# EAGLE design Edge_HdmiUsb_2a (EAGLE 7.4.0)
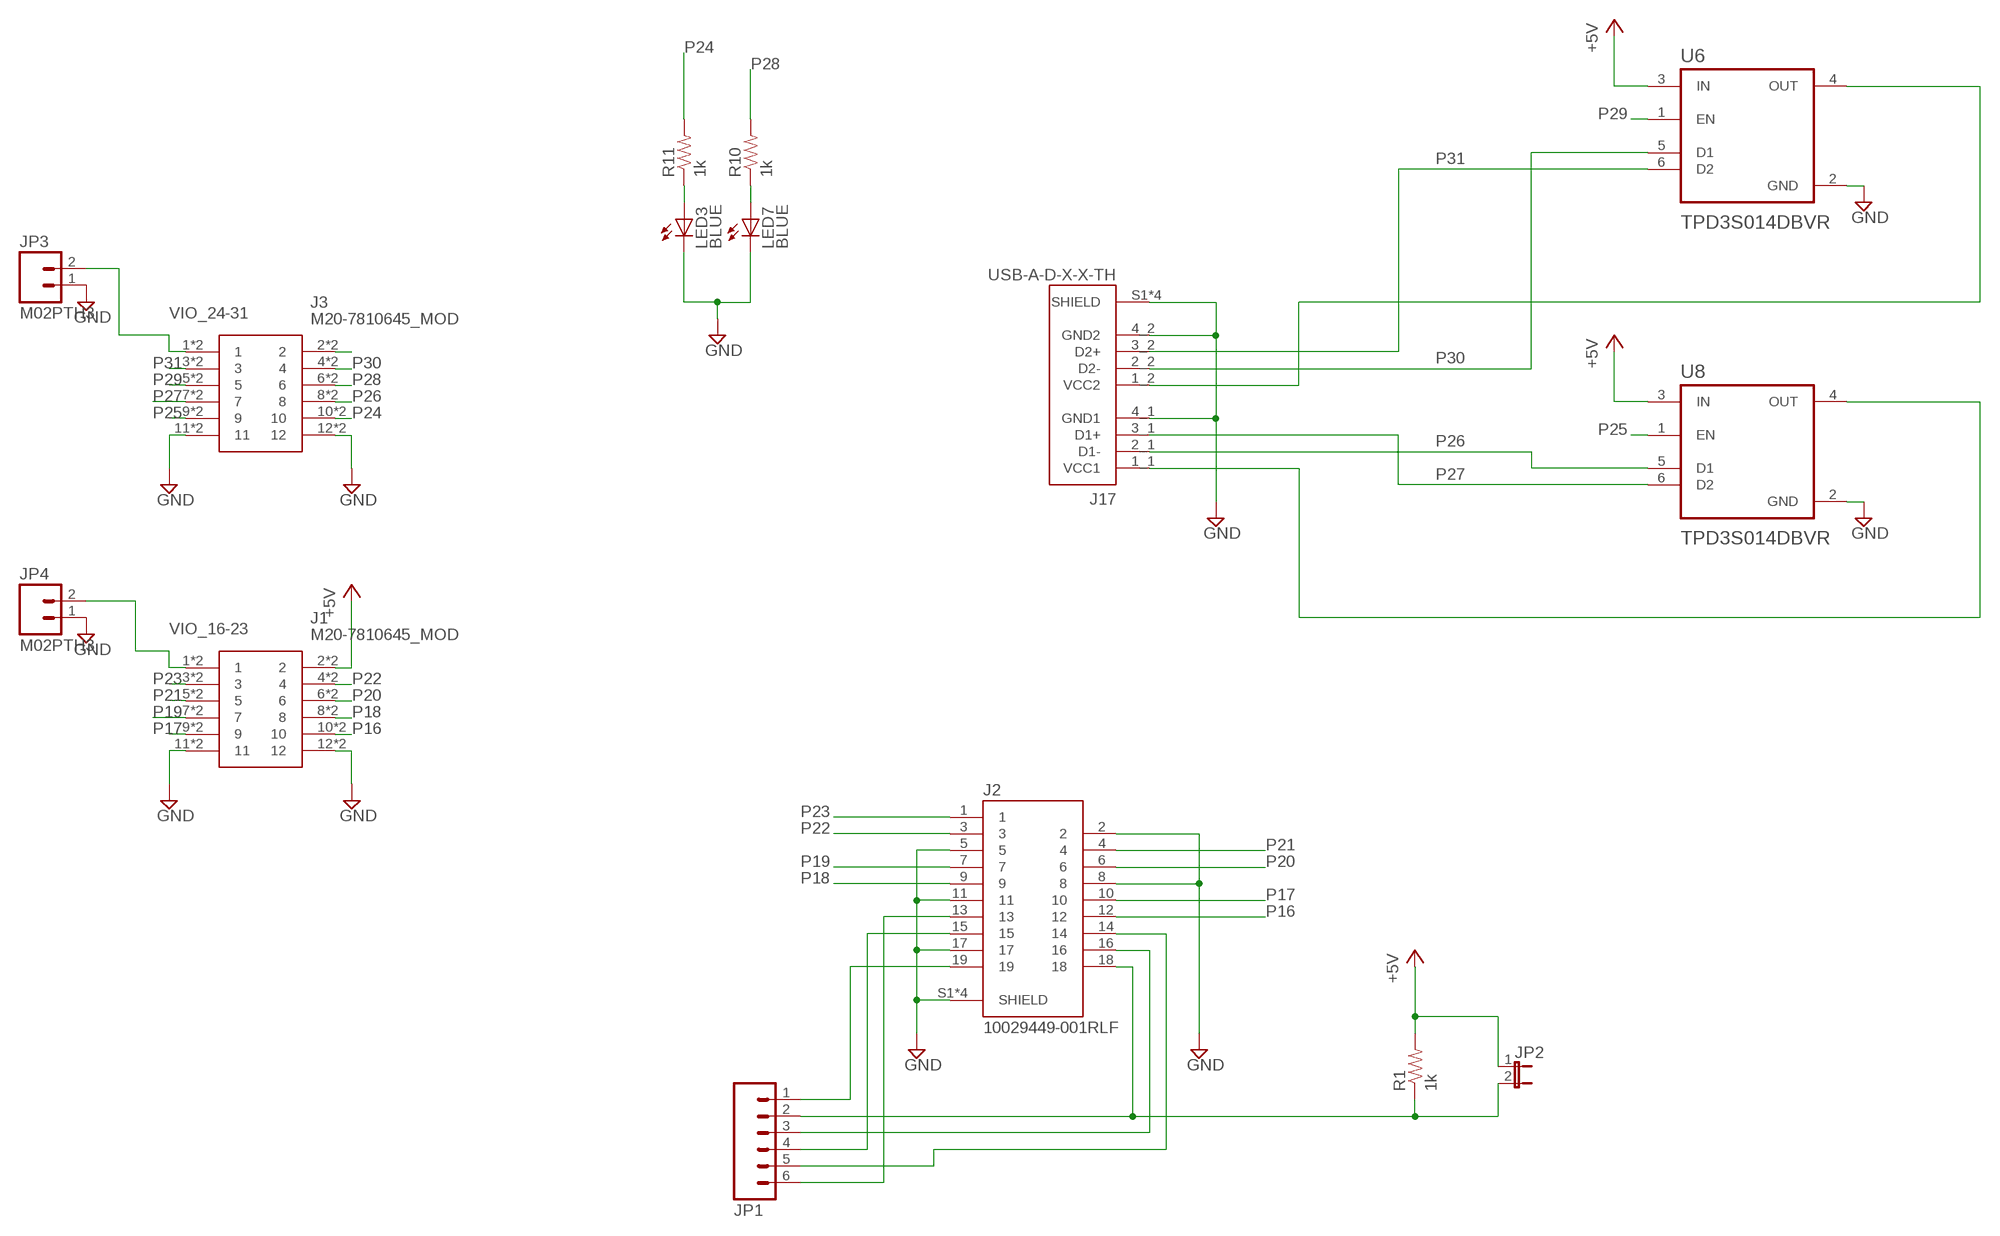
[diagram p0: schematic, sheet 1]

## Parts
J1  M20-7810645_MOD  [M207810645_MOD]
J2  10029449-001RLF  [AMPHENOL_10029449-001RLF]
J3  M20-7810645_MOD  [M207810645_MOD]
J17  USB-A-D-X-X-TH  [SAMTEC_USB-A-D-X-X-TH]
JP1  M06SIP  [1X06]
JP2  JUMPER-2SMD-NO  [SJ_2S-NO]
JP3  M02PTH3  [1X02_LONGPADS]
JP4  M02PTH3  [1X02_LONGPADS]
LED3  BLUE  LEDSML0805  [SML0805]
LED7  BLUE  LEDSML0805  [SML0805]
R1  1k  0.75OHM1/4W1%(0805)  [0805]
R10  1k  0.75OHM1/4W1%(0805)  [0805]
R11  1k  0.75OHM1/4W1%(0805)  [0805]
U6  TPD3S014DBVR  [SOT95P280X145-6N]
U8  TPD3S014DBVR  [SOT95P280X145-6N]

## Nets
+5V: J1.2 J1.2A JP2.1 R1.2 U6.3(IN) U8.3(IN)
GND [power]: J1.11 J1.11A J1.12 J1.12A J2.2 J2.5 J2.8 J2.11 J2.17 J2.S1(SHIELD) J2.S2(SHIELD) J2.S3(SHIELD) J2.S4(SHIELD) J3.11 J3.11A J3.12 J3.12A J17.4_1(GND1) J17.4_2(GND2) J17.S1(SHIELD) J17.S2(SHIELD) J17.S3(SHIELD) J17.S4(SHIELD) JP3.1 JP4.1 LED3.C LED7.C U6.2(GND) U8.2(GND)
N$1: J2.18 JP1.2 JP2.2 R1.1
N$2: J2.16 JP1.3
N$3: J17.1_1(VCC1) U8.4(OUT)
N$4: J2.15 JP1.4
N$5: J2.14 JP1.5
N$6: J3.2 J3.2A
N$8: J2.13 JP1.6
N$19: J2.19 JP1.1
N$23: LED3.A R11.1
N$26: J17.1_2(VCC2) U6.4(OUT)
N$27: LED7.A R10.1
P16: J1.10 J1.10A J2.12
P17: J1.9 J1.9A J2.10
P18: J1.8 J1.8A J2.9
P19: J1.7 J1.7A J2.7
P20: J1.6 J1.6A J2.6
P21: J1.5 J1.5A J2.4
P22: J1.4 J1.4A J2.3
P23: J1.3 J1.3A J2.1
P24: J3.10 J3.10A R11.2
P25: J3.9 J3.9A U8.1(EN)
P26: J3.8 J3.8A J17.2_1(D1-) U8.5(D1)
P27: J3.7 J3.7A J17.3_1(D1+) U8.6(D2)
P28: J3.6 J3.6A R10.2
P29: J3.5 J3.5A U6.1(EN)
P30: J3.4 J3.4A J17.2_2(D2-) U6.5(D1)
P31: J3.3 J3.3A J17.3_2(D2+) U6.6(D2)
VIO_16-23: J1.1 J1.1A JP4.2
VIO_24-31: J3.1 J3.1A JP3.2

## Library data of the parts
J1 J3 = ray2:M20-7810645_MOD: Headers & Wire Housings 6+6 DIL 2.54MM L/P SMT SKT Source: Datasheet; DESCRIPTION: Headers & Wire Housings 6+6 DIL 2.54MM L/P SMT SKT; HEIGHT: 3.7mm; MANUFACTURER_NAME: Harwin; MANUFACTURER_PART_NUMBER: M20-7810645; MOUSER_PART_NUMBER: 855-M20-7810645; MOUSER_PRICE-STOCK: https://www.mouser.co.uk/ProductDetail/Harwin/M20-7810645?qs=k41KVqW3ympKz0jQ%252Bxdz7A%3D%3D
J2 = ray2:10029449-001RLF: Connector, Hdmi Type a, Receptacle, 19 Position, Full Ree; AVAILABILITY: Unavailable; DESCRIPTION: Connector, Hdmi Type a, Receptacle, 19 Position, Full Reel; MF: Amphenol ICC; MP: 10029449-001RLF; PACKAGE: None; PRICE: None
J17 = ray2:USB-A-D-X-X-TH: USB-A (USB TYPE-A), Stacked USB 2.0 Receptacle Connector 8 Position Through Hole, Right Angle Check availability; AVAILABILITY: In Stock; DESCRIPTION: USB-A (USB TYPE-A), Stacked USB 2.0 Receptacle Connector 8 Position Through Hole, Right Angle; MF: Samtec; MP: USB-A-D-F-B-TH; PACKAGE: None; PRICE: None; PURCHASE-URL: https://pricing.snapeda.com/search/part/USB-A-D-F-B-TH/?ref=eda
JP1 = SparkFun-Connectors:M06: Header 6 Standard 6-pin 0.1" header. Use with straight break away headers (SKU : PRT-00116), right angle break away headers (PRT-00553), swiss pins (PRT-00743), machine pins (PRT-00117), and female headers (PRT-00115). Molex polarized connector foot print use with SKU : PRT-08094 with associated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
JP2 = SparkFun-Passives:JUMPER-2: Jumper
JP3 JP4 = SparkFun-Connectors:M02: Standard 2-pin 0.1" header. Use with
LED3 LED7 = led:LED: LED
R1 R10 R11 = SparkFun-Resistors:0.75OHM1/4W1%(0805): RES-08474; PROD_ID: RES-08474; VALUE: 0.75
U6 U8 = ray2:TPD3S014DBVR: Current Limit Switch and D+/D? ESD Protection for USB Host Ports 6-SOT-23 -40 to 85; DESCRIPTION: Current Limit Switch and D+/D? ESD Protection for USB Host Ports 6-SOT-23 -40 to 85; DIGI-KEY_PART_NUMBER: 296-38835-1-ND; DIGI-KEY_PURCHASE_URL: https://www.digikey.com/product-detail/en/texas-instruments/TPD3S014DBVR/296-38835-1-ND/5138398?utm_source=snapeda&utm_medium=aggregator&utm_campaign=symbol; MF: Texas Instruments; MP: TPD3S014DBVR; PACKAGE: SOT-23-6 Texas Instruments

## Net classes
1 power: width 0.254 mm

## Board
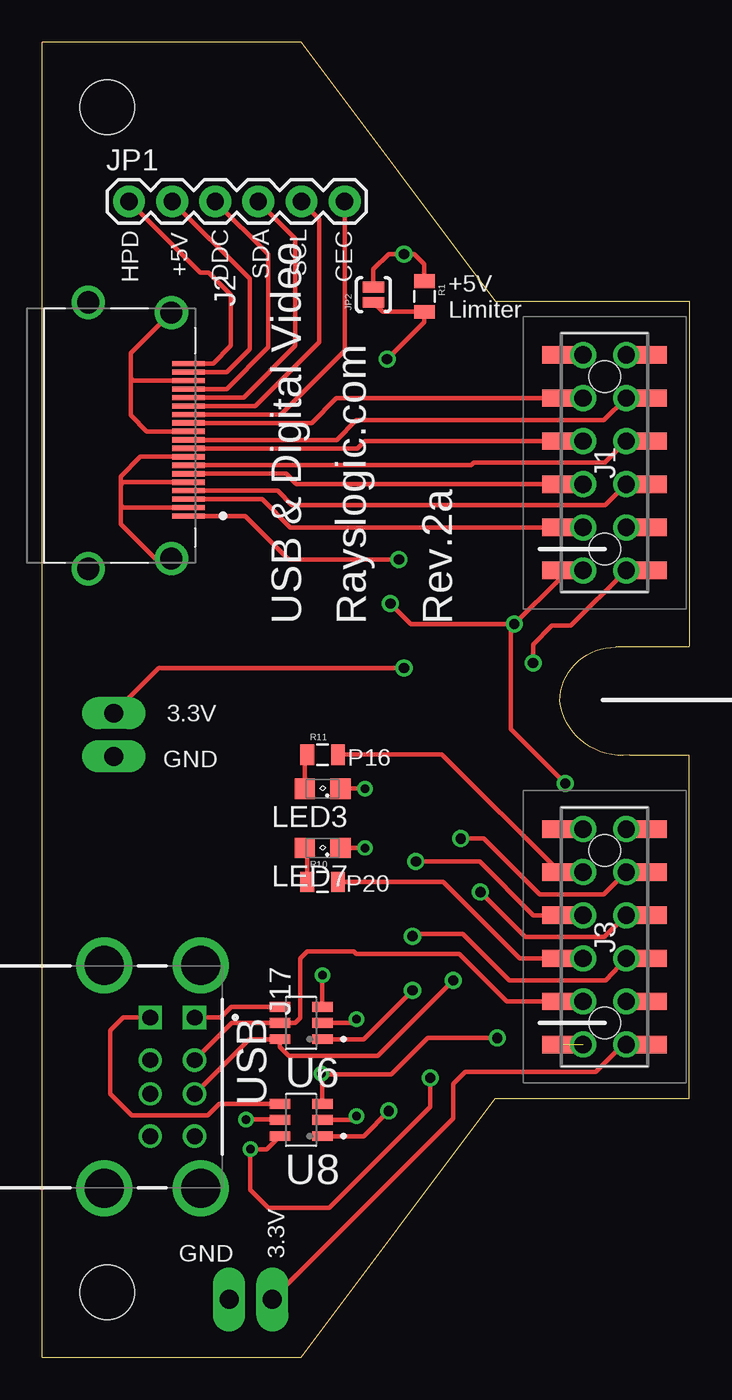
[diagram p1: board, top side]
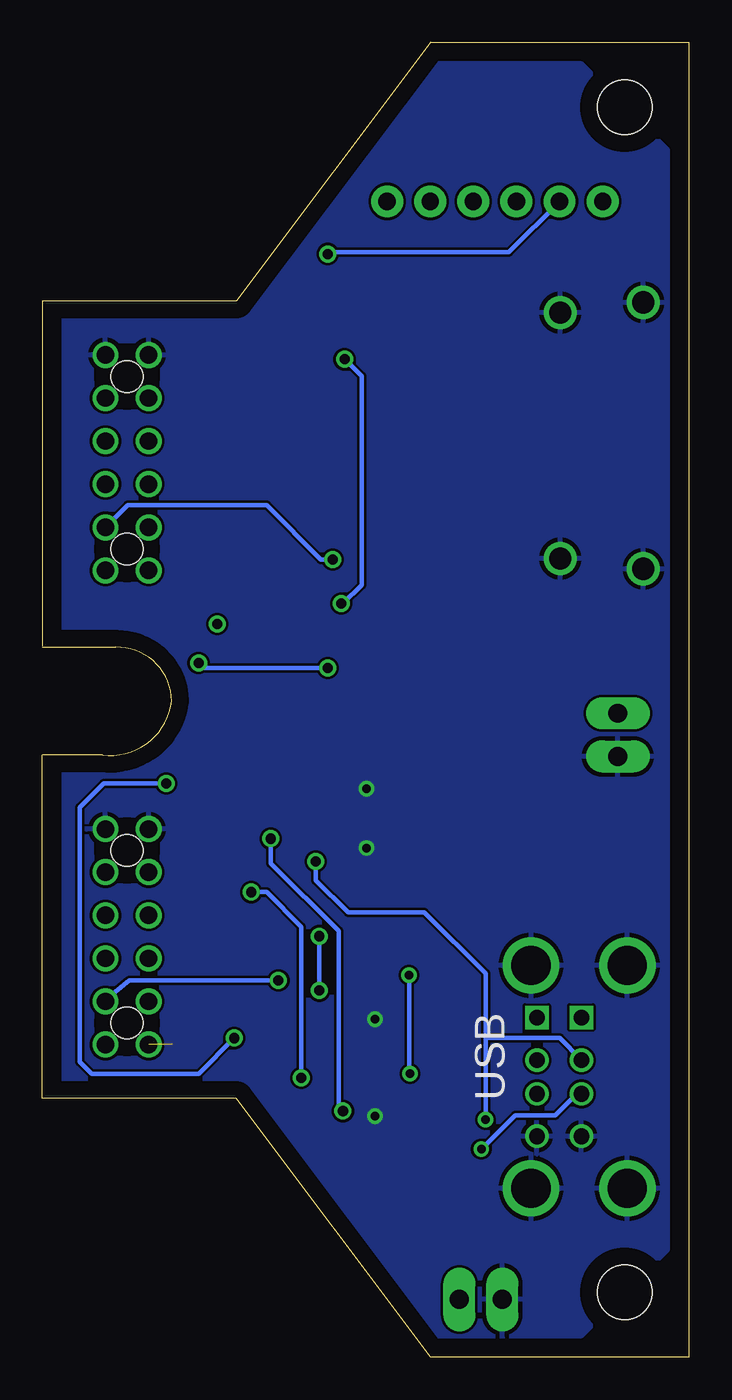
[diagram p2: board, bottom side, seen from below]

Size 38.1 x 77.47 mm. Coordinates in mm from the lower left corner, seen from the top.
Outline: 38.1,41.84 33.78,41.84 arc90 30.48,38.66 arc90 34.56,35.48 38.1,35.48 38.1,15.24 26.67,15.24 15.24,0 0,0 0,77.47 15.24,77.47 26.67,62.23 38.1,62.23 38.1,41.91
Copper layers (1*16): Top 0.035mm / dielectric 1.5mm / Bottom 0.035mm
Design rules "default *": minimum track width 5mil, minimum drill 8mil, track to track 6mil, track to pad 6mil, pad to pad 6mil, via to via 8mil, smd to smd 8mil, copper to edge 40mil, drill to drill 8mil, minimum pad ring 4mil, minimum via ring 8mil, stop-mask expansion 4mil, vias tented up to drill 0mil, thermal gap 10mil
Holes 3.2 mm at 3.81,3.81 3.81,73.66

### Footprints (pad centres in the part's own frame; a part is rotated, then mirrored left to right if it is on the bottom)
M207810645_MOD = smd 1.02 x 2.034: 1 -6.35,-2.656; 2 -6.35,2.656; 3 -3.81,-2.656; 4 -3.81,2.656; 5 -1.27,-2.656; 6 -1.27,2.656; 7 1.27,-2.656; 8 1.27,2.656; 9 3.81,-2.656; 10 3.81,2.656; 11 6.35,-2.656; 12 6.35,2.656 | drill 1.02: 1A -6.35,-1.27; 2A -6.35,1.27; 3A -3.81,-1.27; 4A -3.81,1.27; 5A -1.27,-1.27; 6A -1.27,1.27; 7A 1.27,-1.27; 8A 1.27,1.27; 9A 3.81,-1.27; 10A 3.81,1.27; 11A 6.35,-1.27; 12A 6.35,1.27 | hole 1.85: -5.08,0; 5.08,0
AMPHENOL_10029449-001RLF = smd 0.3 x 1.9: 1 4.75,1; 2 4.25,1; 3 3.75,1; 4 3.25,1; 5 2.75,1; 6 2.25,1; 7 1.75,1; 8 1.25,1; 9 0.75,1; 10 0.25,1; 11 -0.25,1; 12 -0.75,1; 13 -1.25,1; 14 -1.75,1; 15 -2.25,1; 16 -2.75,1; 17 -3.25,1; 18 -3.75,1; 19 -4.25,1 | drill 1.3: S1 7.25,0; S2 -7.25,0; S3 -7.85,-4.9; S4 7.85,-4.9
SAMTEC_USB-A-D-X-X-TH = drill 0.92 square: 1_1 -3.5,0; 1_2 -3.5,2.62 | drill 0.92: 2_1 -1,0; 2_2 -1,2.62; 3_1 1,0; 3_2 1,2.62; 4_1 3.5,0; 4_2 3.5,2.62 | drill 2.3: S1 -6.57,2.97; S2 6.57,2.97; S3 -6.57,-2.71; S4 6.57,-2.71
1X06 = drill 1.016 pad 1.88: 1 0,0; 2 2.54,0; 3 5.08,0; 4 7.62,0; 5 10.16,0; 6 12.7,0
SJ_2S-NO = smd 0.635 x 1.27: 1 -0.45,0; 2 0.45,0
1X02_LONGPADS = drill 1.118 pad 1.88 long: 1 0,0; 2 2.54,0
SML0805 = smd 1.2 x 1.2: A 1.05,0; C -1.05,0
0805 = smd 0.8 x 1.2: 1 -0.9,0; 2 0.9,0
SOT95P280X145-6N = smd 1.21 x 0.58: 1 -1.255,0.95; 2 -1.255,0; 3 -1.255,-0.95; 4 1.255,-0.95; 5 1.255,0; 6 1.255,0.95

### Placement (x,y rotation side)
J1  33.12,52.7 90 top
J2  7.6,54.3 270 top
J3  33.12,24.77 90 top
J17  6.35,16.51 270 top
JP1  5.1,68.1 0 top
JP2  19.5,62.6 90 top
JP3  11,3.4 0 top
JP4  4.2,35.4 90 top
LED3  16.5,33.5 180 top
LED7  16.5,30 180 top
R1  22.5,62.5 270 top
R10  16.5,28 0 top
R11  16.5,35.5 0 top
U6  15.24,19.68 180 top
U8  15.24,13.97 180 top

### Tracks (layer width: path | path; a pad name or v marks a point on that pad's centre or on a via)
+5V  (via drill 0.5, 0.6)
  Top 0.254: U6.3 v16.5,22.5 | U8.3 16.5,16.66 | 16.5,16.66 v16.45,16.7 | 16.5,16.66 20.55,16.66 22.7,18.8 v26.8,18.8 | J1.2A J1.2 | v30.8,33.8 27.6,37 27.6,43 v27.8,43.2 | 30.46,45.86 v27.8,43.2 | JP2.1 20.05,61.6 R1.2 22.5,61 v20.3,58.8 | v20.5,44.4 21.7,43.2 v27.8,43.2
  Top 0.406: J1.2 30.46,45.86
  Bottom 0.254: v16.45,16.7 16.5,16.75 v16.5,22.5 | v30.8,33.8 34.5,33.8 35.9,32.4 35.9,17.4 35.2,16.7 28.9,16.7 v26.8,18.8 | v20.3,58.8 19.3,57.8 19.3,45.5 20.4,44.4 v20.5,44.4
GND  (via drill 0.5)
  Top 0.254: U6.2 18.29,19.68 v18.5,19.91 | U8.2 18.29,13.97 v18.5,14.19 | LED3.C v19,33.5 | LED7.C v19,30 | J3.11A J3.11 | J3.12A J3.12 | J1.11A J1.11 | J1.12A J1.12 | J2.11 6.15,54.55 5.2,55.5 5.2,57.7 | 5.2,57.7 5.2,59.15 J2.S2 | J2.17 5.35,57.55 5.2,57.7 | J2.8 5.75,53.05 4.6,51.9 4.6,51.4 | 4.6,51.4 4.6,50.2 | 4.6,50.2 4.6,49.1 6.65,47.05 J2.S1 | J2.5 4.75,51.55 4.6,51.4 | J2.2 4.75,50.05 4.6,50.2
  pour Bottom (isolate 0.012): 36.83,72.39 36.83,6.35 31.75,1.27 6.35,1.27 1.27,6.35 1.27,71.12 6.35,76.2 33.02,76.2
N$1  (via drill 0.6)
  Top 0.254: J2.18 10.85,58.05 12.2,59.4 12.2,63.54 JP1.2 | R1.1 22.5,64.4 21.9,65 v21.3,65 20.4,65 19.5,64.1 JP2.2 19.5,63.1
  Bottom 0.254: JP1.2 10.64,65.1 21.2,65.1 v21.3,65
N$2
  Top 0.254: J2.16 10.85,57.05 13.3,59.5 13.3,64.98 JP1.3
N$3
  Top 0.254: U8.4 10.42,14.92 9.75,14.25 5.25,14.25 4,15.5 4,19.25 4.76,20.01 J17.1_1
N$4
  Top 0.254: J2.15 11.85,56.55 14.9,59.6 14.9,65.92 JP1.4
N$5
  Top 0.254: J2.14 12.55,56.05 16.3,59.8 16.3,67.06 JP1.5
N$6  (1 unrouted)
N$8
  Top 0.254: J2.13 14.05,55.55 17.8,59.3 JP1.6
N$19
  Top 0.254: J2.19 10.05,58.55 11.1,59.6 11.1,62.6 9.8,63.9 9.3,63.9 JP1.1
N$23
  Top 0.254: R11.1 15.45,35.35 LED3.A
N$26
  Top 0.254: U6.4 11.13,20.64 10.51,20.01 J17.1_2
N$27
  Top 0.254: LED7.A 15.6,29.85 R10.1
P16
  Top 0.254: J1.10A J1.10 17.32,56.52 15.85,55.05 J2.12
P17
  Top 0.254: J1.9 J1.9A 33.07,55.2 18.5,55.2 17.35,54.05 J2.10
P18
  Top 0.254: J1.8A J1.8 18.98,53.98 18.55,53.55 J2.9
P19
  Top 0.254: J1.7 J1.7A 33.11,52.7 25.4,52.7 25.25,52.55 J2.7
P20
  Top 0.254: J1.6A J1.6 14.96,51.44 14.35,52.05 J2.6
P21
  Top 0.254: J1.5 J1.5A 33.15,50.2 14.7,50.2 13.85,51.05 J2.4
P22
  Top 0.254: J1.4A J1.4 14.61,48.9 12.95,50.55 J2.3
P23  (via drill 0.6)
  Top 0.254: J1.3A J1.3 | v21,47 14.5,47 11.95,49.55 J2.1
  Bottom 0.254: J1.3A 33.08,50.2 24.9,50.2 21.7,47 v21,47
P24
  Top 0.254: J3.10A J3.10 23.54,35.5 R11.2
P25  (via drill 0.6)
  Top 0.254: v24.65,30.55 26,30.55 29.3,27.25 33.06,27.25 J3.9A J3.9 | v20.4,14.5 18.92,13.02 U8.1
  Bottom 0.254: v24.65,30.55 24.65,29.1 20.65,25.1 20.65,14.75 v20.4,14.5
P26  (via drill 0.5, 0.6)
  Top 0.254: U8.5 13.96,14 v12,14 | v22,29.2 25.75,29.2 28.91,26.04 J3.8 J3.8A
  Bottom 0.254: 12,18.8 12,22.6 15.6,26.2 20.1,26.2 22,28.1 v22,29.2 | 12,18.8 v12,14 | J17.2_1 7.64,18.8 12,18.8
P27  (via drill 0.5, 0.6)
  Top 0.254: U8.6 13.21,12.25 v12.25,12.25 12.25,9.85 13.3,8.8 16.9,8.8 22.85,14.75 v22.85,16.45 | v25.8,27.4 28.45,24.75 33.1,24.75 J3.7A J3.7
  Bottom 0.254: v12.25,12.25 10.25,14.25 7.9,14.25 6.64,15.51 J17.3_1 | v25.8,27.4 24.9,27.4 22.85,25.35 v22.85,16.45
P28
  Top 0.254: R10.2 23.6,28 28.11,23.5 J3.6 J3.6A
P29  (via drill 0.6)
  Top 0.254: J3.5 J3.5A 33.19,22.2 27.5,22.2 24.75,24.95 21.95,24.95 v21.8,24.8 | U6.1 18.93,18.73 v21.8,21.6
  Bottom 0.254: v21.8,21.6 v21.8,24.8
P30
  Top 0.254: J17.2_2 11.14,19.68 U6.5 14.88,19.68 15.2,20 15.2,23.5 15.6,23.9 18.35,23.9 18.5,23.75 24.55,23.75 27.34,20.95 J3.4 J3.4A
P31  (via drill 0.6)
  Top 0.254: J17.3_2 12.2,18.73 U6.6 13.98,18.27 14.5,17.75 19.75,17.75 v24.2,22.2 | J3.3 J3.3A
  Bottom 0.254: J3.3A 34.31,21.09 33,22.2 v24.2,22.2
VIO_16-23  (via drill 0.6)
  Top 0.254: J1.1 J1.1A 31.13,43.1 30,43.1 28.9,42 v28.9,40.9 | v21.3,40.6 6.86,40.6 JP4.2
  Bottom 0.254: v28.9,40.9 28.6,40.6 v21.3,40.6
VIO_24-31
  Top 0.254: J3.1 J3.1A 34.22,18.41 32.6,16.8 24.9,16.8 24.2,16.1 24.2,14.06 JP3.2

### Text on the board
tPlace: Rev.2A / Making skinny so can work with Eval/Edge / Disconnecting lower 5V for WX | HPD | +5V | DDC | SDA | SCL | CEC | +5V / Limiter | USB & Digital Video | Rayslogic.com | Rev.2a | 3.3V | P16 | GND | P20 | USB | GND | 3.3V
bPlace: USB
